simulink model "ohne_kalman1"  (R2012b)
settings: Solver=ode45  StartTime=0.0  StopTime=10.0  RelTol=1e-3
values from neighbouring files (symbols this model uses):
  a1 = a1{:}    [ohne_kalman_1.m]    (also in coulomb_10.m = subplot(311), plot(t, vy-vb); coulomb_11.m = subplot(311), plot(t, vy-vb); coulomb_2.m = subplot(311),  plot(t, y1); coulomb_3.m = subplot(311),  plot(t, y1))
  b1 = b1{:}    [ohne_kalman_1.m]
  D = 0    [aktiv_tilger_1.m]    (also in aktiv_tilger_12.m; aktiv_tilger_3.m = 2000; aktiv_tilger_31.m; beobachter_1.m)
  dt = 0.01    [aktiv_tilger_1.m]    (also in aktiv_tilger_12.m; aktiv_tilger_2.m; beobachter_1.m; beobachter_2.m)
  I = 2000    [aktiv_tilger_1.m]    (also in aktiv_tilger_12.m; aktiv_tilger_3.m = 0; aktiv_tilger_31.m = 0; fuellstnd_2.m = 0.0225)
  P = 0    [aktiv_tilger_1.m]    (also in aktiv_tilger_12.m; aktiv_tilger_3.m; aktiv_tilger_31.m; fuellstnd_2.m = 0.09)
  vnd = 1e-4    (= 0.0001)    [kalman_1.m]    (also in kalman_10.m; kalman_11.m; kalman_12.m; kalman_13.m = 0.01)
  vny = 1e-6    (= 1e-06)    [kalman_1.m]    (also in kalman_10.m; kalman_11.m = ', num2str(vny),' )']); kalman_12.m = ', num2str(vny),' )']); kalman_13.m = ', num2str(vny),' )']))
libraries: simulink x1

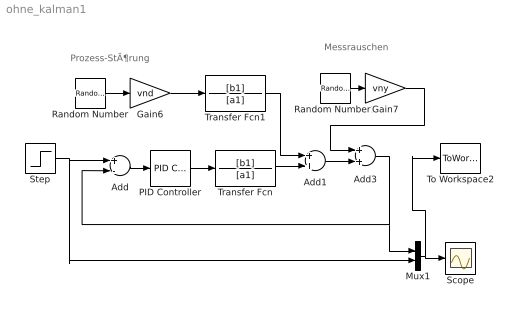
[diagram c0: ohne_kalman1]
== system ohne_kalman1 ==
  note: Prozess-StÃ¶rung
  note: Messrauschen
  Add : Sum  Inputs=+-
  Add1 : Sum
  Add3 : Sum
  Gain6 : Gain  Gain=vnd
  Gain7 : Gain  Gain=vny
  Mux1 : Mux  Inputs=2
  PID Controller : simulink/Continuous/PID Controller  Controller=PID  TimeDomain=Continuous-time  SampleTime=1  IntegratorMethod=Forward Euler  FilterMethod=Forward Euler  Form=Parallel  P=P  I=I  D=D  N=100  InitialConditionSource=internal  InitialConditionForIntegrator=0  InitialConditionForFilter=0  ExternalReset=none  LimitOutput=off  UpperSaturationLimit=inf  LowerSaturationLimit=-inf  LinearizeAsGain=on  AntiWindupMode=none  Kb=1  TrackingMode=off  Kt=1  PParamMin=[]  PParamMax=[]  IParamMin=[]  IParamMax=[]  DParamMin=[]  DParamMax=[]  NParamMin=[]  NParamMax=[]  KbParamMin=[]  KbParamMax=[]  KtParamMin=[]  KtParamMax=[]  POutMin=[]  POutMax=[]  IOutMin=[]  IOutMax=[]  DOutMin=[]  DOutMax=[]  NOutMin=[]  NOutMax=[]  KbOutMin=[]  KbOutMax=[]  KtOutMin=[]  KtOutMax=[]  IntegratorOutMin=[]  IntegratorOutMax=[]  FilterOutMin=[]  FilterOutMax=[]  SumOutMin=[]  SumOutMax=[]  SumI1OutMin=[]  SumI1OutMax=[]  SumI2OutMin=[]  SumI2OutMax=[]  SumI3OutMin=[]  SumI3OutMax=[]  SumDOutMin=[]  SumDOutMax=[]  SaturationOutMin=[]  SaturationOutMax=[]  IntegratorContinuousStateAttributes=''  IntegratorStateMustResolveToSignalObject=off  IntegratorRTWStateStorageClass=Auto  FilterContinuousStateAttributes=''  FilterStateMustResolveToSignalObject=off  FilterRTWStateStorageClass=Auto
  Random Number : RandomNumber  SampleTime=dt*10
  Random Number1 : RandomNumber  Seed=18967  SampleTime=dt*10
  Scope : Scope
  Step : Step  SampleTime=0
  To Workspace2 : ToWorkspace  VariableName=y  SaveFormat=Structure With Time
  Transfer Fcn : TransferFcn  Numerator=[b1]  Denominator=[a1]
  Transfer Fcn1 : TransferFcn  Numerator=[b1]  Denominator=[a1]
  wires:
  Add/1 -> PID Controller/1
  Transfer Fcn/1 -> Add1/2
  Transfer Fcn1/1 -> Add1/1
  Random Number/1 -> Gain6/1
  Gain6/1 -> Transfer Fcn1/1
  Random Number1/1 -> Gain7/1
  Gain7/1 -> Add3/1
  Add1/1 -> Add3/2
  PID Controller/1 -> Transfer Fcn/1
  Add3/1 -> Mux1/1, Add/2
  Mux1/1 -> To Workspace2/1, Scope/1
  Step/1 -> Mux1/2, Add/1
